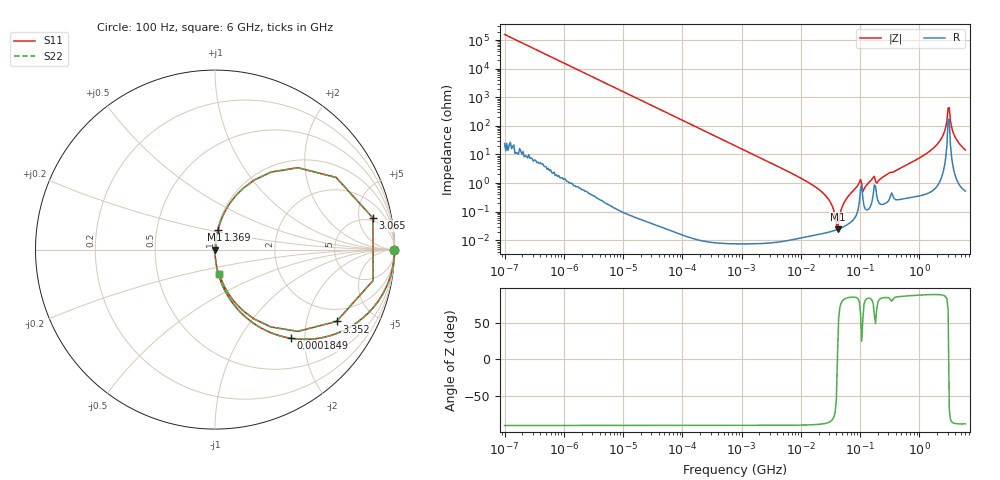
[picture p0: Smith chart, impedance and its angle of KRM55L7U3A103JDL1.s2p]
!Murata Part Number: KRM55L7U3A103JDL1
!These Parameters are Measured in Series Mode Connection
!Data Generated on Jan 08, 2026
!  o--ll--o
!Port1  Port2
!  o------o
!Operation Temp=25[degC], DC Bias Voltage=0[V]
!Freq. Start=100[Hz] Stop=6[GHz] 401[Steps]
# Hz S RI R 50
!Freq.(Hz) S11(Real) S11(Imag) S21(Real) S21(Imag) S12(Real) S12(Imag) S22(Real) S22(Imag)
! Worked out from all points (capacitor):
!   401 points, 100 Hz to 6 GHz, reference 50 ohm
!   read as one part in series: C = 10.1 nF near 109 Hz
!   lowest |Z| = 24 mohm at 41.66 MHz (marker M1)
!   series resonance near 41.53 MHz, so ESL is about 1.5 nH
!   S11 on the Smith chart (normalised r, x): 100 Hz: open; 184.9 kHz: 1.00, -1.70; 1.369 GHz: 1.01, +0.23; 3.065 GHz: 4.27, +7.73; 3.352 GHz: 1.44, -3.03; 6 GHz: 1.01, -0.29
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100  1 -0.000635  5e-07 0.000635  5e-07 0.000635  1 -0.000635
2008  0.9998 -0.0127  0.000163 0.0127  0.000163 0.0127  0.9998 -0.0127
40335  0.9385 -0.2402  0.0615 0.2402  0.0615 0.2402  0.9385 -0.2402
184852  0.4209 -0.4936  0.5791 0.4936  0.5791 0.4936  0.4209 -0.4936
774597  0.0398 -0.1953  0.9602 0.1953  0.9602 0.1953  0.0398 -0.1953
1.555665e7  0.000219 -0.00869  0.9998 0.00869  0.9998 0.00869  0.000219 -0.00869
2.911731e7  0.000197 -0.00276  0.9998 0.00276  0.9998 0.00276  0.000197 -0.00276
4.165952e7  0.000238 2.52e-05  0.9998 -2.52e-05  0.9998 -2.52e-05  0.000238 2.52e-05
5.699437e7  0.000328 0.00251  0.9997 -0.00251  0.9997 -0.00251  0.000328 0.00251
9.326766e7  0.00131 0.00866  0.9987 -0.00866  0.9987 -0.00866  0.00131 0.00866
1.220122e8  0.0013 0.00716  0.9987 -0.00716  0.9987 -0.00716  0.0013 0.00716
1.596157e8  0.0025 0.0136  0.9975 -0.0136  0.9975 -0.0136  0.0025 0.0136
1.996653e8  0.00255 0.0109  0.9974 -0.0109  0.9974 -0.0109  0.00255 0.0109
3.124326e8  0.00319 0.0222  0.9968 -0.0222  0.9968 -0.0222  0.00319 0.0222
1.369159e9  0.0168 0.111  0.9832 -0.111  0.9832 -0.111  0.0168 0.111
2.34314e9  0.1206 0.3057  0.8794 -0.3057  0.8794 -0.3057  0.1206 0.3057
2.802721e9  0.4619 0.4562  0.5381 -0.4562  0.5381 -0.4562  0.4619 0.4562
3.065283e9  0.8795 0.1766  0.1205 -0.1766  0.1205 -0.1766  0.8795 0.1766
3.352442e9  0.6772 -0.4  0.3228 0.4  0.3228 0.4  0.6772 -0.4
3.666503e9  0.3115 -0.431  0.6885 0.431  0.6885 0.431  0.3115 -0.431
4.193612e9  0.1173 -0.3014  0.8827 0.3014  0.8827 0.3014  0.1173 -0.3014
6e9  0.0248 -0.1383  0.9752 0.1383  0.9752 0.1383  0.0248 -0.1383
